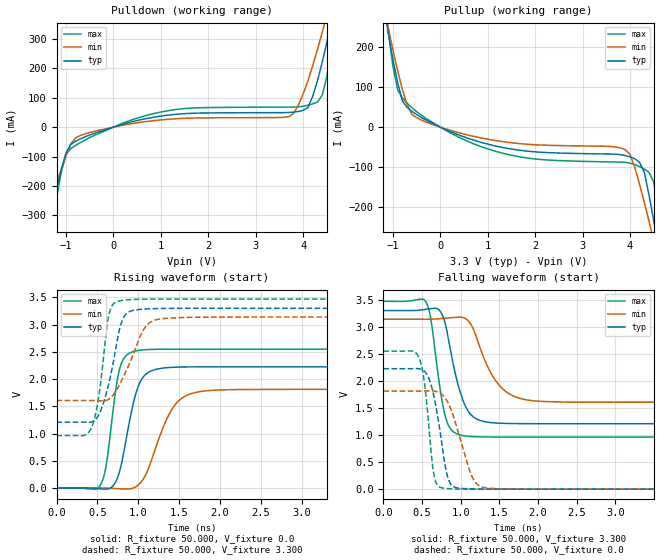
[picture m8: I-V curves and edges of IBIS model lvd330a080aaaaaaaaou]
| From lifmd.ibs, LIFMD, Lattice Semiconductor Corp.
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|   Model lvd330a080aaaaaaaaou
[Model] lvd330a080aaaaaaaaou
Model_type Output
Polarity   Non-Inverting
Vmeas =  1.650V
Cref =  0.0F
Rref =  1.000M
Vref =  0.0V
C_comp   5.000pF   4.000pF   5.500pF
[Temperature Range]   25.000   0.125k   -40.000
[Voltage Range]   3.300V   3.140V   3.470V
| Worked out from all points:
|   slope of the pulldown table from 0 to 0.495 V, typ, clamps not added: 22.2 ohm
|   slope of the pullup table from 0 to 0.495 V, typ, clamps not added: 20.5 ohm
|   rising waveform, R_fixture 50.000, V_fixture 0.0: 20-80 % time 185ps typ, 288ps min, 134ps max; typ from 0 V to 2.23 V
|   rising waveform, R_fixture 50.000, V_fixture 3.300: 20-80 % time 178ps typ, 261ps min, 124ps max; typ from 1.21 V to 3.3 V
|   falling waveform, R_fixture 50.000, V_fixture 3.300: 20-80 % time 207ps typ, 307ps min, 149ps max; typ from 3.3 V to 1.21 V
|   falling waveform, R_fixture 50.000, V_fixture 0.0: 20-80 % time 154ps typ, 231ps min, 107ps max; typ from 2.23 V to 0 V
[Pulldown]
|Voltage   I(typ)   I(min)   I(max)
-3.3V     -1.776A    -1.307A    -2.431A
-1.5V     -423.6mA   -342.8mA   -538.4mA
-1.4V     -351.5mA   -291.1mA   -437.4mA
-1.3V     -280.6mA   -240.3mA   -338.1mA
-1V       -86.97mA   -97.65mA   -93.09mA
-600mV    -33.08mA   -22.8mA    -43.84mA
1.2V      41.65mA    27.29mA    57.19mA
3.7V      49.78mA    35.79mA    67.98mA
4.1V      66.56mA    157.4mA    74.46mA
4.5V      288.6mA    381.2mA    171.9mA
4.7V      439.3mA    507.4mA    377.8mA
6.6V      2.168A     1.924A     3.534A
[Pullup]
|Voltage   I(typ)   I(min)   I(max)
-3.3V     2.151A     1.834A     3.789A
-1.1V     235.9mA    249.4mA    241.7mA
-900mV    110.8mA    140.5mA    92.9mA
-700mV    49.1mA     55.83mA    59.51mA
-500mV    31.42mA    23.54mA    38.71mA
1.3V      -50.32mA   -35.76mA   -64.44mA
3.8V      -68.46mA   -51.76mA   -86.99mA
4V        -74.06mA   -67.96mA   -89.6mA
4.2V      -87.28mA   -141.6mA   -98.17mA
4.5V      -232.6mA   -283.4mA   -137mA
4.7V      -369.1mA   -384.5mA   -298.2mA
6.6V      -1.78A     -1.393A    -2.261A
[Ramp]
| variable   typ   min   max
dV/dt_r   1.335/0.193n   1.087/0.297n   1.530/0.140n
dV/dt_f   1.255/0.212n   0.920/0.311n   1.505/0.156n
R_load = 50.000
[Rising Waveform]
R_fixture= 50.000
V_fixture= 0.0
V_fixture_min= 0.0
V_fixture_max= 0.0
|time   V(typ)   V(min)   V(max)
0s        0V         0V         0V
536ps     -16.16mV   759.6uV    52.64mV
606ps     -21.46mV   -2.929mV   401.5mV
725ps     115.9mV    -11.53mV   1.805V
775ps     321mV      -14.23mV   2.204V
999ps     1.864V     52.71mV    2.526V
1.129ns   2.127V     373.8mV    2.543V
1.414ns   2.215V     1.45V      2.55V
1.764ns   2.225V     1.772V     2.55V
10ns      2.225V     1.812V     2.55V
[Rising Waveform]
R_fixture= 50.000
V_fixture= 3.300
V_fixture_min= 3.140
V_fixture_max= 3.470
|time   V(typ)   V(min)   V(max)
0s        1.209V     1.607V     962.5mV
332ps     1.209V     1.607V     963mV
426ps     1.21V      1.607V     1.102V
516ps     1.34V      1.604V     1.673V
641ps     1.928V     1.633V     3.18V
789ps     3.016V     1.951V     3.442V
874ps     3.224V     2.222V     3.456V
1.074ns   3.286V     2.93V      3.468V
1.334ns   3.298V     3.115V     3.47V
10ns      3.3V       3.14V      3.47V
[Falling Waveform]
R_fixture= 50.000
V_fixture= 3.300
V_fixture_min= 3.140
V_fixture_max= 3.470
|time   V(typ)   V(min)   V(max)
0s        3.3V       3.14V      3.47V
548ps     3.323V     3.139V     3.464V
612ps     3.334V     3.141V     3.159V
730ps     3.297V     3.15V      1.883V
801ps     3.05V      3.159V     1.342V
1.038ns   1.61V      3.168V     988mV
1.184ns   1.314V     2.882V     969.4mV
1.489ns   1.22V      1.935V     963mV
1.938ns   1.21V      1.634V     962.5mV
10ns      1.209V     1.607V     962.5mV
[Falling Waveform]
R_fixture= 50.000
V_fixture= 0.0
V_fixture_min= 0.0
V_fixture_max= 0.0
|time   V(typ)   V(min)   V(max)
0s        2.225V     1.812V     2.55V
464ps     2.224V     1.812V     2.415V
532ps     2.176V     1.814V     1.949V
651ps     1.728V     1.813V     287.9mV
772ps     678.2mV    1.729V     19.5mV
833ps     216.8mV    1.605V     10.3mV
894ps     59.61mV    1.393V     5.855mV
1.146ns   4.774mV    233.2mV    594.5uV
1.315ns   1.376mV    26.01mV    127.7uV
10ns      0V         0V         0V
